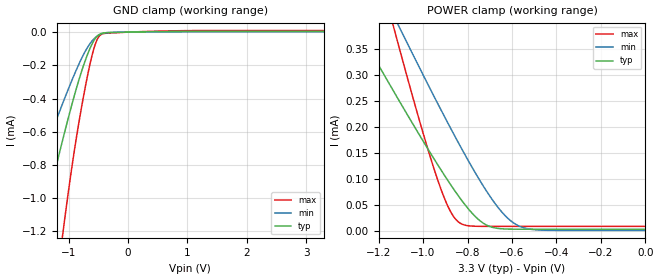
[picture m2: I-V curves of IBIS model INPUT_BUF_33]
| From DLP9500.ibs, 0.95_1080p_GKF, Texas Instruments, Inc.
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[Model]   INPUT_BUF_33
Model_type  Input
Vinl=0.70
Vinh=2.00
| variable   typ   min   max
C_comp   0.26pF   0.21pF   0.30pF
[Temperature Range]   40   125   -40
| Ambient temperature   25   110   -40
[Voltage range]   3.3   3   3.6
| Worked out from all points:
|   GND clamp passes 1 mA (typ) near -1.34 V on its own axis
|   POWER clamp passes 1 mA (typ) near -2.09 V on its own axis
[GND Clamp]
| INPUT_BUF_33
|   Voltage   I(typ)   I(min)   I(max)
-3.3V     -4.113mA   -2.669mA   -8.127mA
-1.925V   -1.896mA   -1.236mA   -3.704mA
-1.87V    -1.809mA   -1.18mA    -3.531mA
-1.465V   -1.184mA   -775.7uA   -2.279mA
-1.1V     -645.9uA   -426.9uA   -1.213mA
-890mV    -362.3uA   -242uA     -677.9uA
-730mV    -179.3uA   -121uA     -346.8uA
-580mV    -53.41uA   -42.57uA   -103.8uA
-525mV    -25.82uA   -25.32uA   -47.45uA
-475mV    -11.95uA   -14.38uA   -19.98uA
565mV     3.13uA     1.571uA    6.56uA
3.3V      4.206uA    1.925uA    9.709uA
[POWER Clamp]
| INPUT_BUF_33
|   Voltage   I(typ)   I(min)   I(max)
-3.3V     1.941mA    2.381mA    4.062mA
-1.3V     392.9uA    560.1uA    663.2uA
-1.13V    266.8uA    411.3uA    387.8uA
-1.11V    252.2uA    394uA      356.2uA
-1.095V   241.3uA    381uA      332.7uA
-935mV    128.4uA    245.7uA    99.8uA
-885mV    95.4uA     204.9uA    45.32uA
-840mV    67.54uA    169uA      17.96uA
-720mV    13.44uA    80.87uA    9.748uA
-630mV    4.693uA    29.87uA    9.722uA
-565mV    4.253uA    9.73uA     9.721uA
-48.03fV  4.206uA    1.92uA     9.713uA
